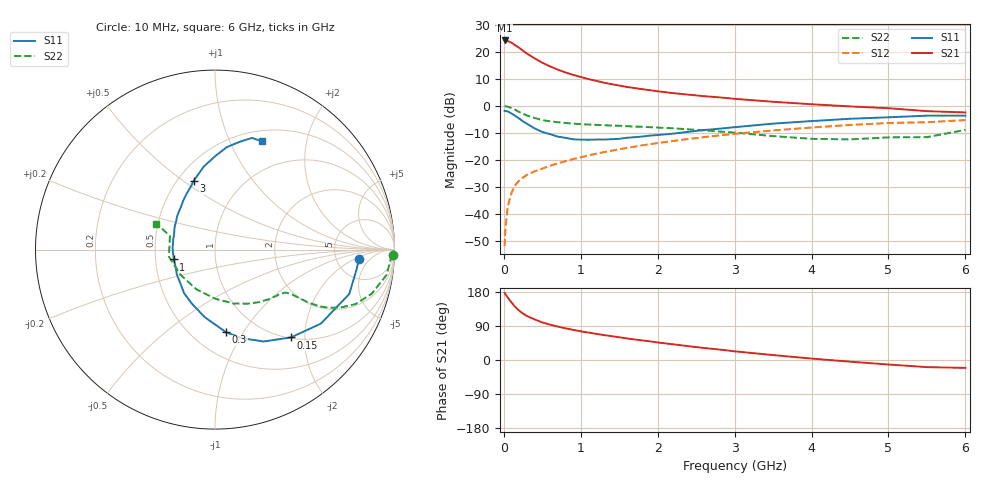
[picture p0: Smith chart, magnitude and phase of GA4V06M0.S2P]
! Infineon Technologies  Discrete & RF Semiconductors
! BF775
! Si NPN RF Bipolar Junction Transistor in SOT23
! VCE = 4 V  IC = 6 mA
! Common Emitter S-Parameters:  May  1996
# GHz  S  MA  R  50
!  f  S11  S21  S12  S22
! GHz  MAG  ANG  MAG  ANG  MAG  ANG  MAG  ANG
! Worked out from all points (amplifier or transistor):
!   36 points, 10 MHz to 6 GHz, reference 50 ohm
!   highest |S21| = 24.2 dB at 10 MHz (marker M1)
!   |S21| within 3 dB of that: start of sweep to 211.5 MHz
!   unconditionally stable (mu >= 1): 749.7 MHz to 3.336 GHz
!   at 250 MHz: K = 0.54, MSG = 23.5 dB, |S12| = -26.6 dB
!   at 1.4 GHz: K = 1.12, MAG = 10.2 dB, |S12| = -16.6 dB
!   at 6 GHz: K = 0.95, MSG = 1.4 dB, |S12| = -5.3 dB
!   S11 on the Smith chart (normalised r, x): 10 MHz: 8.44, -2.47; 150 MHz: 1.02, -1.71; 300 MHz: 0.72, -0.84; 1 GHz: 0.62, -0.07; 3 GHz: 0.60, +0.55; 6 GHz: 0.62, +1.33
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0.01  0.8033 -3.7  16.25 176.9  0.0025 88.5  0.9916 -1.7
0.02  0.7974 -7.5  15.94 173.6  0.0051 83.8  0.9794 -3.4
0.05  0.7878 -18.3  15.84 165.1  0.0134 80.4  0.9662 -8.4
0.1  0.7197 -35.0  14.8 151.6  0.0245 73.4  0.9064 -15.8
0.15  0.6465 -49.2  13.18 139.6  0.0342 66.6  0.8392 -21.2
0.2  0.5793 -62.1  11.84 130.1  0.0412 62.9  0.7686 -24.9
0.25  0.5143 -73.4  10.45 122.3  0.047 60.5  0.7074 -27.2
0.3  0.4652 -82.3  9.28 116.3  0.0524 58.7  0.6624 -28.5
0.4  0.3805 -98.7  7.571 107.0  0.0611 57.6  0.5934 -29.6
0.5  0.328 -113.0  6.278 99.2  0.0684 57.9  0.5434 -29.9
0.6  0.298 -125.3  5.379 93.4  0.0772 58.4  0.5151 -30.1
0.7  0.2681 -136.3  4.695 88.2  0.0857 58.9  0.4966 -30.2
0.8  0.2546 -146.6  4.159 83.7  0.094 59.1  0.4802 -30.6
1  0.2358 -166.5  3.417 75.7  0.111 60.0  0.4564 -31.7
1.1  0.2347 -174.9  3.13 72.4  0.1203 60.0  0.4493 -32.8
1.6  0.2554 152.2  2.231 57.0  0.1657 58.3  0.4186 -39.2
2.2  0.3046 128.5  1.717 41.4  0.2229 54.3  0.3827 -49.9
3  0.4013 107.2  1.346 22.9  0.3018 46.3  0.3183 -70.8
3.5  0.4671 97.7  1.187 13.0  0.349 40.4  0.2741 -89.5
4.5  0.5747 83.4  0.974 -4.4  0.4409 27.6  0.2381 -144.1
5.5  0.6556 71.7  0.795 -18.8  0.4966 12.7  0.2623 163.2
6  0.657 66.6  0.753 -20.8  0.5427 8.6  0.3572 156.0
